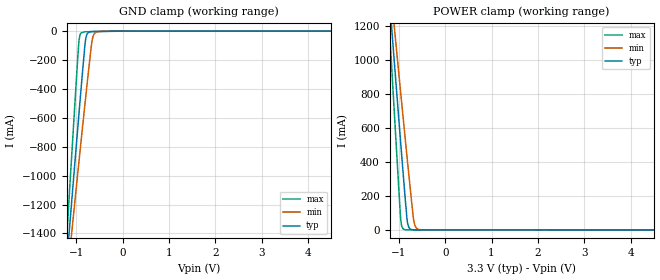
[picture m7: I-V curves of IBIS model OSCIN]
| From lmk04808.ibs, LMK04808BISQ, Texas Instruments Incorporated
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|   Model   OSCIN
[Model]   OSCIN
Model_type   Input
Vinl = 1.6
Vinh = 2.0
|   typ   min   max
|   (nom PVT)   (fast PVT)   (slow PVT)
C_comp   3.0731pF   2.9226pF   3.0881pF
[Voltage Range]   3.3   3.15   3.45
[Temperature Range]   45   125   -40
[Power Clamp Reference]   3.3   3.15   3.45
[GND Clamp Reference]   0   0   0
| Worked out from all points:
|   GND clamp passes 1 mA (typ) near -0.20 V on its own axis
|   POWER clamp passes 1 mA (typ) near -0.68 V on its own axis
[GND Clamp]
|   Voltage   I(typ)   I(min)   I(max)
-3.3V     -9.963A    -8.491A    -12.66A
-1.32V    -2.04A     -2.091A    -2.021A
-1.142V   -1.34A     -1.526A    -1.079A
-1.023V   -877.2mA   -1.152A    -459.2mA
-953.7mV  -610mA     -934.7mA   -108.7mA
-933.9mV  -534.4mA   -872.9mA   -46.34mA
-894.3mV  -384.9mA   -750mA     -12.02mA
-815.1mV  -95.84mA   -507.3mA   -4.927mA
-785.4mV  -35.96mA   -418mA     -4.556mA
-656.7mV  -3.174mA   -58.84mA   -3.718mA
-557.7mV  -2.235mA   -5.072mA   -3.163mA
6.59V     0A         0A         0A
[POWER Clamp]
|   Voltage   I(typ)   I(min)   I(max)
-3.3V     8.842A     7.525A     11.27A
-1.221V   1.422A     1.543A     1.272A
-1.053V   833.9mA    1.069A     482.4mA
-963.6mV  525.7mA    818.8mA    76.27mA
-943.8mV  457.8mA    763.5mA    30.11mA
-904.2mV  323.4mA    653.4mA    5.406mA
-825mV    65.85mA    435.5mA    896.9uA
-805.2mV  32.99mA    381.8mA    811.9uA
-676.5mV  989.2uA    53.24mA    603.9uA
-636.9mV  589.2uA    17.47mA    481.7uA
-577.5mV  369.7uA    3.486mA    365.3uA
6.59V     0A         0A         0A
